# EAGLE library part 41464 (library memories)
DRAM 64K x 4 bits
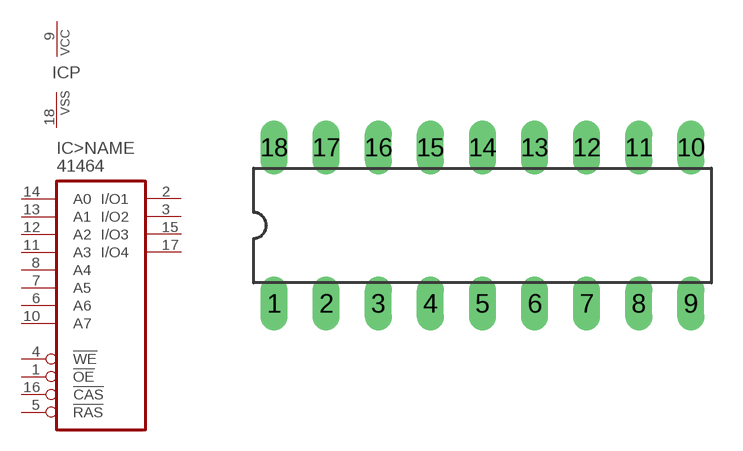
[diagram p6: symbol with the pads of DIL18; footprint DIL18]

Designator prefix IC; gates >NAME=DRAM64KX4 P=VCCVSS

## 41464  [DIL18]
1  >NAME:!OE  in
2  >NAME:I/O1
3  >NAME:I/O2
4  >NAME:!WE  in
5  >NAME:!RAS  in
6  >NAME:A6  in
7  >NAME:A5  in
8  >NAME:A4  in
9  P:VCC  pwr
10  >NAME:A7  in
11  >NAME:A3  in
12  >NAME:A2  in
13  >NAME:A1  in
14  >NAME:A0  in
15  >NAME:I/O3
16  >NAME:!CAS  in
17  >NAME:I/O4
18  P:VSS  pwr

## Footprint DIL18 (pad centres in mm)
Dual In Line
drill 0.813 long: 1 -10.16,-3.81; 2 -7.62,-3.81; 3 -5.08,-3.81; 4 -2.54,-3.81; 5 0,-3.81; 6 2.54,-3.81; 7 5.08,-3.81; 8 7.62,-3.81; 9 10.16,-3.81; 10 10.16,3.81; 11 7.62,3.81; 12 5.08,3.81; 13 2.54,3.81; 14 0,3.81; 15 -2.54,3.81; 16 -5.08,3.81; 17 -7.62,3.81; 18 -10.16,3.81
